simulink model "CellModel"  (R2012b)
settings: Solver=ode3  StartTime=0.0  StopTime=70  FixedStep=0.1  RelTol=1e-3
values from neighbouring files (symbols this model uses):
  Ct = 2700    [PowerInputValidationTest.m]    (also in SimulationScript.m; SCmodel.m)
  I = zeros(1,length(t))    [SimulationScript.m]
  Q = 2*3600    (= 7200)    [PowerInputValidationTest.m]    (also in SimulationScript.m; SCmodel.m)
  Rs = 0.008    [PowerInputValidationTest.m]    (also in SimulationScript.m; SCmodel.m)
  Rt = 0.011    [PowerInputValidationTest.m]    (also in SimulationScript.m; SCmodel.m)
  SOC = [0 0.1 0.2 0.3 0.4 0.5 0.6 0.7 0.8 0.9 1]    [PowerInputValidationTest.m]    (also in SimulationScript.m; SCmodel.m; int_series.m = 1:1:101)
  SOC_0 = 0.5    [PowerInputValidationTest.m]    (also in SimulationScript.m; SCmodel.m)
  V = [2.25 3.2 3.25 3.25 3.3 3.3 3.3 3.35 3.35 3.35 3.75]    [PowerInputValidationTest.m]    (also in SimulationScript.m; SCmodel.m; int_series.m = [2.000; 2.760; 2.885; 2.963; 3.020; 3.066; 3.103; 3.136; 3.1)
undefined symbols (not defined in the file or in its folder): InitialSOC

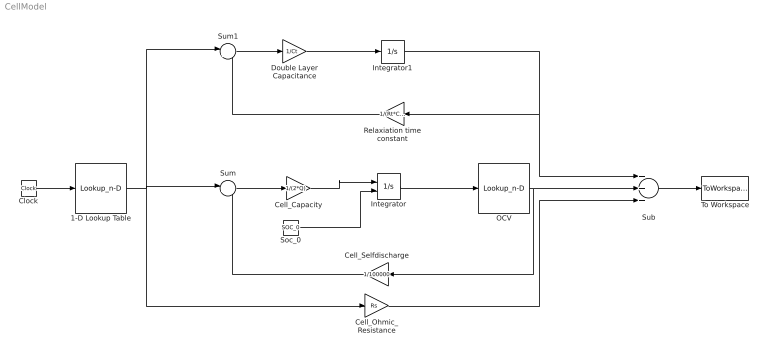
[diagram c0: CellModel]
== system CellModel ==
  1-D Lookup Table : Lookup_n-D  NumberOfTableDimensions=1  BreakpointsForDimension1=t  Table=I  RndMeth=Simplest
  Cell_Capacity : Gain  Gain=1/(2*Q)
  Cell_Ohmic_Resistance : Gain  Gain=Rs
  Cell_Selfdischarge : Gain  Gain=1/100000
  Clock : Clock
  Double Layer Capacitance : Gain  Gain=1/Ct
  Integrator : Integrator  InitialConditionSource=external  InitialCondition=InitialSOC
  Integrator1 : Integrator
  OCV : Lookup_n-D  NumberOfTableDimensions=1  BreakpointsForDimension1=SOC  Table=V  RndMeth=Simplest
  Relaxiation time constant : Gain  Gain=1/(Rt*Ct)
  Soc_0 : Constant  Value=SOC_0
  Sub : Sum  Inputs=+++
  Sum : Sum  Inputs=|+-
  Sum1 : Sum  Inputs=|+-
  To Workspace : ToWorkspace  VariableName=voltage  SampleTime=-1  SaveFormat=Structure With Time
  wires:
  Integrator/1 -> OCV/1
  OCV/1 -> Cell_Selfdischarge/1, Sub/2
  1-D Lookup Table/1 -> Sum1/1, Cell_Ohmic_Resistance/1, Sum/1
  Cell_Capacity/1 -> Integrator/1
  Cell_Selfdischarge/1 -> Sum/2
  Integrator1/1 -> Relaxiation time constant/1, Sub/1
  Relaxiation time constant/1 -> Sum1/2
  Cell_Ohmic_Resistance/1 -> Sub/3
  Sub/1 -> To Workspace/1
  Sum/1 -> Cell_Capacity/1
  Double Layer Capacitance/1 -> Integrator1/1
  Sum1/1 -> Double Layer Capacitance/1
  Soc_0/1 -> Integrator/2
  Clock/1 -> 1-D Lookup Table/1
